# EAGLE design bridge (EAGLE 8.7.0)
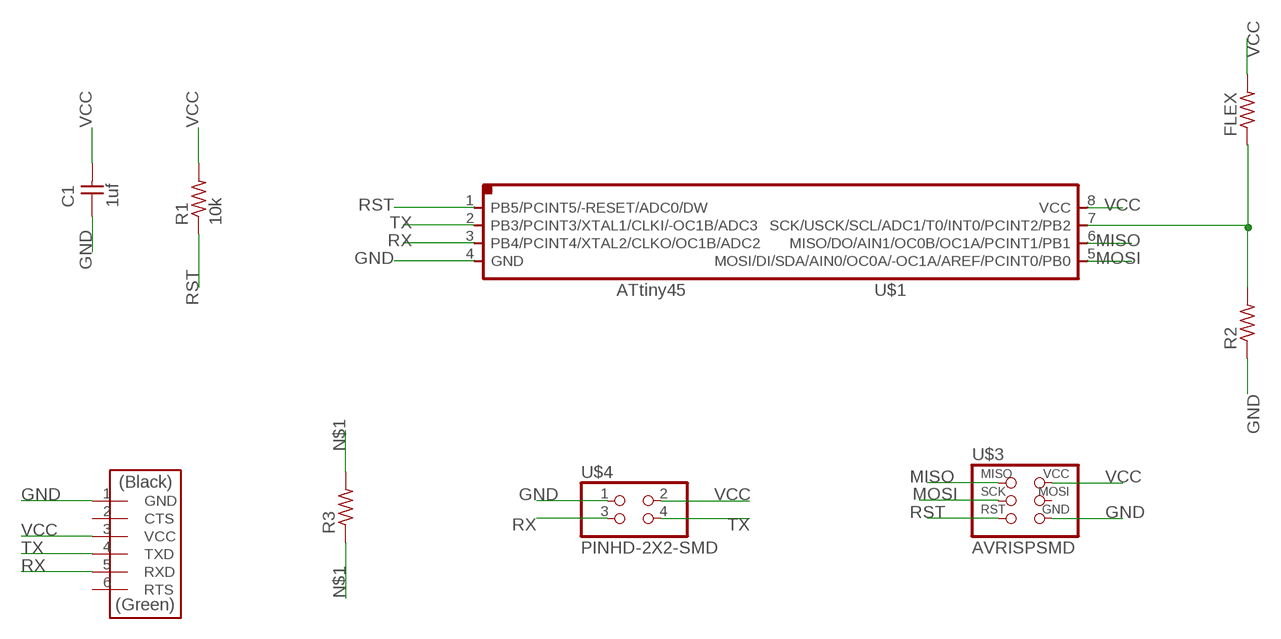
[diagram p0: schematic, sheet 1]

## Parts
C1  1uf  CAP-UNPOLARIZEDFAB  [C1206FAB]
FLEX  RES-US1206FAB  [R1206FAB]
R1  10k  RES-US1206FAB  [R1206FAB]
R2  RES-US1206FAB  [R1206FAB]
R3  RES-US1206FAB  [R1206FAB]
U$1  ATTINY45SI  [SOIC8]
U$2  FTDI-SMD-HEADER  [1X06SMD]
U$3  AVRISPSMD  [2X03SMD]
U$4  PINHD-2X2-SMD  [2X02SMD]

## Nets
GND: C1.1 R2.1 U$1.4(GND) U$2.1(GND) U$3.6(GND) U$4.1
MISO: U$1.6(MISO/DO/AIN1/OC0B/OC1A/PCINT1/PB1) U$3.1(MISO)
MOSI: U$1.5(MOSI/DI/SDA/AIN0/OC0A/-OC1A/AREF/PCINT0/PB0) U$3.3(SCK)
N$1: FLEX.1 R2.2 R3.1 R3.2 U$1.7(SCK/USCK/SCL/ADC1/T0/INT0/PCINT2/PB2)
RST: R1.1 U$1.1(PB5/PCINT5/-RESET/ADC0/DW) U$3.5(RST)
RX: U$1.3(PB4/PCINT4/XTAL2/CLKO/OC1B/ADC2) U$2.5(RXD) U$4.3
TX: U$1.2(PB3/PCINT3/XTAL1/CLKI/-OC1B/ADC3) U$2.4(TXD) U$4.4
VCC: C1.2 FLEX.2 R1.2 U$1.8(VCC) U$2.3(VCC) U$3.2(VCC) U$4.2
Unconnected: U$2.2(CTS) U$2.6(RTS) U$3.4(MOSI)

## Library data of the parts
C1 = fab:CAP-UNPOLARIZED
FLEX R1-R3 = fab:RES-US: Resistor (US Symbol)
U$1 = ng:ATTINY45
U$2 = fab:FTDI-SMD-HEADER
U$3 = fab:AVRISP
U$4 = fab:PINHD-2X2-SMD

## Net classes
0 default: width 0.4 mm, drill 0.4 mm, clearance 0.4 mm

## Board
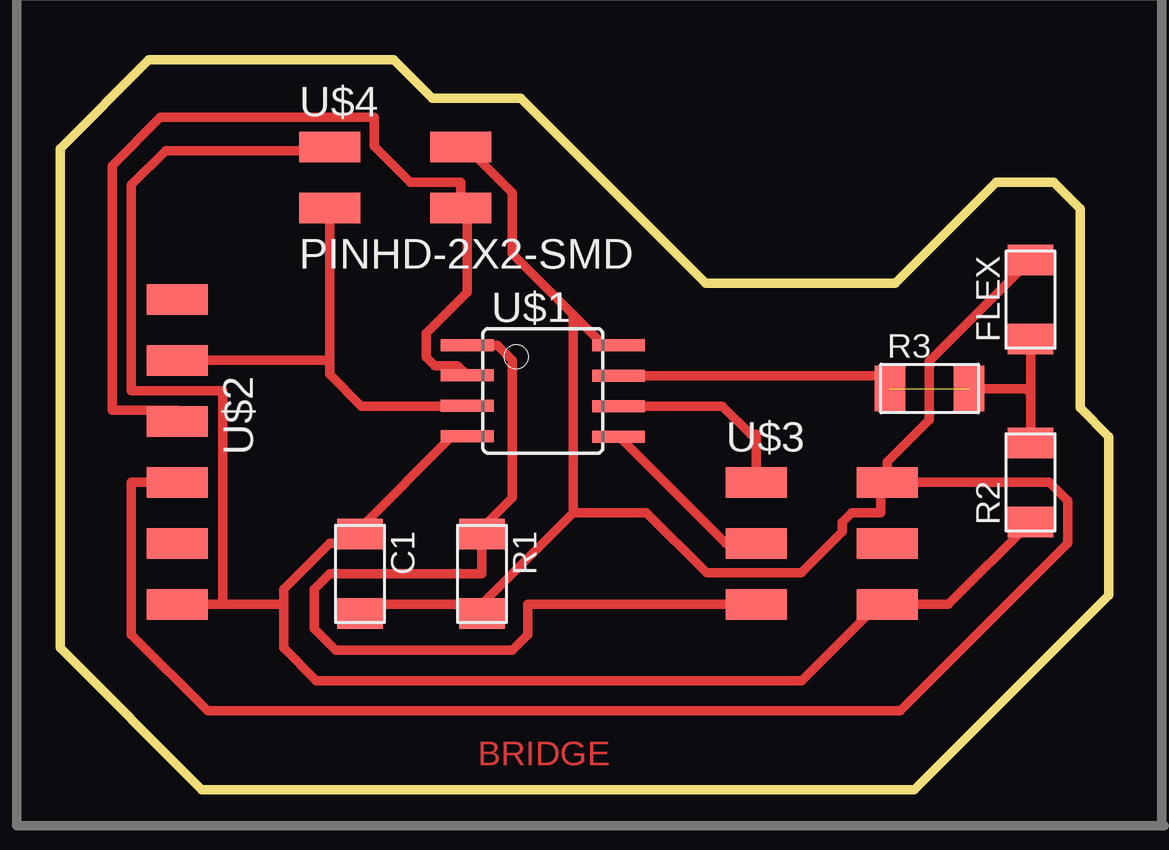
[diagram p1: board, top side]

Size 43.7 x 30.4 mm. Coordinates in mm from the lower left corner, seen from the top.
Outline: 0,5.9 0,26.7 3.7,30.4 13.9,30.4 15.5,28.8 19.2,28.8 26.9,21.1 34.8,21.1 39,25.3 41.4,25.3 42.5,24.2 42.5,15.9 43.7,14.7 43.7,8.1 35.6,0 5.9,0 0,5.9
Copper layers (1*16): Top 0.035mm / dielectric 1.5mm / Bottom 0.035mm
Design rules "default *": minimum track width 0.4mm, minimum drill 0.35mm, track to track 0.4mm, track to pad 6mil, pad to pad 6mil, via to via 0.4mm, smd to smd 6mil, copper to edge 40mil, drill to drill 6mil, minimum pad ring 10mil, minimum via ring 8mil, stop-mask expansion 4mil, vias tented up to drill 0mil, thermal gap 10mil

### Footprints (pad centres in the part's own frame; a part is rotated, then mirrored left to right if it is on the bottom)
C1206FAB = smd 1.27 x 1.905: 1 -1.651,0; 2 1.651,0
R1206FAB = smd 1.27 x 1.905: 1 -1.651,0; 2 1.651,0
SOIC8 = smd 0.5 x 2.2: 1 -1.905,-3.154; 2 -0.645,-3.154; 3 0.625,-3.154; 4 1.895,-3.154; 5 1.905,3.154; 6 0.635,3.154; 7 -0.635,3.154; 8 -1.905,3.154
1X06SMD = smd 2.54 x 1.27: 1 0,6.35; 2 0,3.81; 3 0,1.27; 4 0,-1.27; 5 0,-3.81; 6 0,-6.35
2X03SMD = smd 2.54 x 1.27: 1 -2.54,2.54; 2 2.92,2.54; 3 -2.54,0; 4 2.92,0; 5 -2.54,-2.54; 6 2.92,-2.54
2X02SMD = smd 2.54 x 1.27: 1 -2.54,1.27; 2 2.92,1.27; 3 -2.54,-1.27; 4 2.92,-1.27

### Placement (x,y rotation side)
C1  12.5,8.99 270 top
FLEX  40.44,20.42 90 top
R1  17.58,8.99 270 top
R2  40.44,12.8 90 top
R3  36.23,16.71 0 top
U$1  20.12,16.61 270 top
U$2  4.88,14.07 180 top
U$3  31.55,10.26 0 top
U$4  13.77,25.5 0 top

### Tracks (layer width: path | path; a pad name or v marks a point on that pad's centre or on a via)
GND
  Top 0.4: U$1.4 16.95,14.71 16.31,14.71 12.5,10.89 C1.1 12.5,10.26 11.23,10.26 9.33,8.36 9.33,7.72 | 9.33,7.72 6.79,7.72 | 6.79,7.72 U$2.1 | 6.79,7.72 6.79,16.61 2.97,16.61 2.97,25.2 4.4,26.62 11.09,26.62 U$4.1 | 9.33,7.72 9.33,5.9 10.68,4.54 30.91,4.54 34.09,7.72 U$3.6 37.01,7.72 R2.1
MISO
  Top 0.4: U$1.6 27.6,15.97 28.78,14.8 29.01,14.8 U$3.1
MOSI
  Top 0.4: U$3.3 27.74,10.26 23.3,14.71 U$1.5
N$1  (1 unrouted)
  Top 0.4: 40.44,16.5 FLEX.1 40.44,19.15 | 40.44,16.5 R2.2 | U$1.7 34.04,17.25 R3.1 | R3.2 40.23,16.71 40.44,16.5
RST
  Top 0.4: U$1.1 18.21,18.52 18.85,17.88 18.85,12.16 17.58,10.89 R1.1 17.58,8.99 11.23,8.99 10.6,8.36 10.6,6.7 11.48,5.81 18.85,5.81 19.48,6.45 19.48,7.72 U$3.5
RX
  Top 0.4: U$4.3 11.23,17.88 | 11.23,17.88 11.23,17.3 12.56,15.97 16.95,15.97 U$1.3 | 11.23,17.88 U$2.5
TX
  Top 0.4: U$2.4 4.88,15.81 2.17,15.81 2.17,26 4.18,28.01 13.1,28.01 13.1,26.8 14.6,25.3 16.69,25.3 U$4.4 16.97,23.95 16.97,20.71 15.27,19.01 15.27,18.02 15.62,17.67 16.56,17.67 U$1.2
VCC
  Top 0.4: 17.58,7.72 12.5,7.72 C1.2 | 21.39,19.79 18.85,22.33 18.85,24.87 16.95,26.77 U$4.2 | 21.39,19.79 22.66,18.52 U$1.8 | 21.39,11.53 17.58,7.72 | 21.39,19.79 21.39,11.53 | 17.58,7.72 R1.2 | 40.44,21.69 FLEX.2 36.21,17.85 36.21,15.41 34.47,13.66 U$3.2 | U$2.3 2.97,12.8 2.97,6.45 6.15,3.27 35,3.27 41.99,10.26 41.99,12.03 41.22,12.8 U$3.2 | 34.09,12.8 34.2,12.8 | 34.2,12.8 U$3.2 | 34.2,12.8 34.2,11.53 32.99,11.53 32.6,11.14 32.6,10.74 30.88,9.03 26.94,9.03 24.44,11.53 21.39,11.53

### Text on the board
Top: BRIDGE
